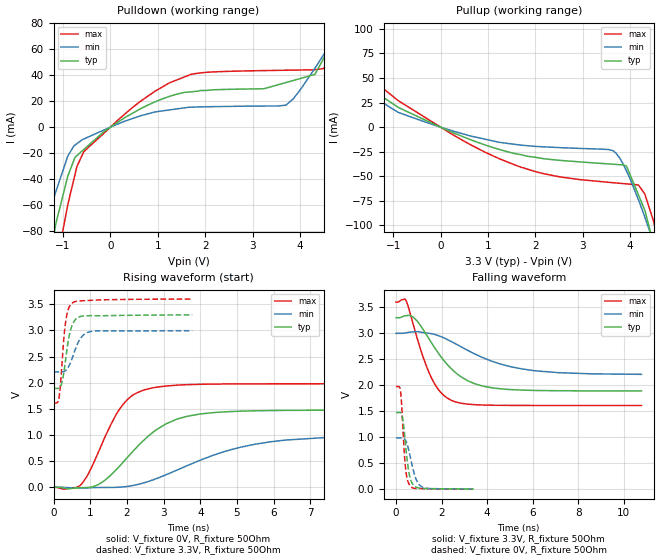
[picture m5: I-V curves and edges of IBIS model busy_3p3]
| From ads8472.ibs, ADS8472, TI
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|   busy_3p3 Model
[Model]   busy_3p3
Model_type   Output
Polarity   Non-Inverting
Vmeas = 1.65
Vref = 1.65
Cref = 5pF
Rref = 50
|   typ   min   max
|   (nom PVT)   (Fast PVT)   (slow PVT)
|C_comp from frequency method(F=1MHz)
|Average
|C_comp   8.471e-12   7.455e-12   1.492e-11
|ON state : BUFFER OUTPUT TURNED HIGH
|C_comp   8.471e-12   7.455e-12   1.492e-11
|OFF state: BUFFER OUTPUT TURNED LOW
|C_comp   5.617e-12   4.472e-12   6.741e-12
|C_comp from L-C Tank method(L=1nH)
|Resonant Frequency(Hz)   3.46e9   3.94e9   3.1e9
C_comp   2.118e-12   1.633e-12  2.638e-12
| Where nom  PVT is Nominal Process,  3.3V,  30C
|   Fast PVT is Strong Process,   3.6V,  -40C
|   Slow PVT is Weak Process,   3V,  90C
[Voltage Range]   3.3   3   3.6
|Ambient Temperature   25   85   -40
|Junction Temperature
[Temperature Range]   30   90   -40
[Pullup Reference]   3.3   3   3.6
[Pulldown Reference]   0   0   0
[Power Clamp Reference]   3.3   3   3.6
[GND Clamp Reference]   0   0   0
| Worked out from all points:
|   slope of the pulldown table from 0 to 0.495 V, typ, clamps not added: 44 ohm
|   slope of the pullup table from 0 to 0.495 V, typ, clamps not added: 48.8 ohm
|   falling waveform, V_fixture 3.3V, R_fixture 50Ohm: 20-80 % time 1.55ns typ, 2.51ns min, 984ps max; typ from 3.3 V to 1.89 V
|   rising waveform, V_fixture 0V, R_fixture 50Ohm: 20-80 % time 1.34ns typ, 2.32ns min, 849ps max; typ from 0 V to 1.48 V
|   rising waveform, V_fixture 3.3V, R_fixture 50Ohm: 20-80 % time 193ps typ, 275ps min, 144ps max; typ from 1.89 V to 3.3 V
|   falling waveform, V_fixture 0V, R_fixture 50Ohm: 20-80 % time 232ps typ, 335ps min, 168ps max; typ from 1.48 V to 0.005 V
[Pulldown]
|   Voltage   I(typ)   I(min)   I(max)
-3.3V     -554.4mA   -390.5mA   -764.5mA
-1.357V   -116.1mA   -76.09mA   -164.7mA
-1.141V   -72.84mA   -48.65mA   -106mA
-897.6mV  -37.49mA   -22.12mA   -59.52mA
-745.8mV  -23.17mA   -13.73mA   -36.37mA
-561.6mV  -17.21mA   -9.126mA   -19mA
1.246V    23.65mA    13.24mA    34.04mA
3.702V    34.28mA    16.89mA    43.81mA
4.316V    40.58mA    45.23mA    44.14mA
4.662V    63.94mA    64.84mA    54.8mA
5.28V     106.2mA    96.98mA    107.1mA
6.6V      169.4mA    151.6mA    195.9mA
[Pullup]
|   Voltage   I(typ)   I(min)   I(max)
-3.3V     137.8mA    121.9mA    160.8mA
-2.837V   119.1mA    103.6mA    142.1mA
-2.235V   90.94mA    78.66mA    107.7mA
-1.415V   40.88mA    35.74mA    47.28mA
-897mV    20.21mA    15.12mA    27.04mA
1.645V    -27.56mA   -17.98mA   -39.87mA
3.639V    -37.74mA   -24mA      -56.56mA
3.924V    -39.56mA   -44.57mA   -57.75mA
4.18V     -69.29mA   -74.17mA   -59.12mA
4.468V    -114.1mA   -113.5mA   -91.64mA
4.655V    -152.9mA   -141.4mA   -133.4mA
6.6V      -597.1mA   -466.9mA   -733.5mA
[Ramp]
R_load = 50
|   typ   min   max
dV/dt_r   0.887057/1.33633e-09   0.591584/2.32234e-09   1.18783/8.48849e-10
dV/dt_f   0.845912/1.55421e-09   0.475367/2.52494e-09   1.19342/9.8449e-10
[Falling Waveform]
V_fixture = 3.3V
V_fixture_min = 3V
V_fixture_max = 3.6V
R_fixture = 50Ohm
|   Time   V(typ)   V(min)   V(max)
0s        3.3V       3V         3.6V
430ps     3.338V     3.009V     3.639V
880ps     3.259V     3.031V     2.98V
1.19ns    3.073V     3.014V     2.544V
1.55ns    2.823V     2.993V     2.149V
1.97ns    2.552V     2.937V     1.861V
2.47ns    2.3V       2.832V     1.704V
3.65ns    2.004V     2.563V     1.623V
5.52ns    1.908V     2.316V     1.613V
10.77ns   1.891V     2.211V     1.611V
[Rising Waveform]
V_fixture = 0V
V_fixture_min = 0V
V_fixture_max = 0V
R_fixture = 50Ohm
|   Time   V(typ)   V(min)   V(max)
0s        1.018nV    1.181nV    912pV
760ps     -7.584mV   -18.63mV   59.4mV
1.25ns    63.56mV    -3.895mV   715.2mV
1.79ns    396.6mV    1.69mV     1.483V
2.13ns    661.2mV    29.56mV    1.746V
2.49ns    919.4mV    90.64mV    1.866V
3.07ns    1.214V     240.2mV    1.937V
3.64ns    1.357V     413mV      1.962V
5.9ns     1.467V     868.2mV    1.978V
10.75ns   1.477V     982.1mV    1.98V
[Rising Waveform]
V_fixture = 3.3V
V_fixture_min = 3V
V_fixture_max = 3.6V
R_fixture = 50Ohm
|   Time   V(typ)   V(min)   V(max)
0s        1.89V      2.207V     1.611V
150ps     1.894V     2.207V     1.717V
190ps     1.923V     2.206V     1.971V
240ps     2.035V     2.206V     2.456V
330ps     2.444V     2.232V     3.162V
420ps     2.87V      2.319V     3.434V
520ps     3.119V     2.491V     3.528V
740ps     3.267V     2.852V     3.564V
1.02ns    3.28V      2.978V     3.574V
3.78ns    3.296V     2.994V     3.598V
[Falling Waveform]
V_fixture = 0V
V_fixture_min = 0V
V_fixture_max = 0V
R_fixture = 50Ohm
|   Time   V(typ)   V(min)   V(max)
0s        1.477V     987.8mV    1.976V
200ps     1.475V     988.1mV    1.88V
240ps     1.452V     988.7mV    1.678V
300ps     1.341V     988.4mV    1.207V
410ps     909.3mV    949.9mV    445.4mV
480ps     606.4mV    878.8mV    224.9mV
610ps     236.9mV    658.2mV    71.75mV
870ps     43.2mV     206.6mV    16.54mV
1.16ns    16.81mV    42.14mV    13.2mV
3.41ns    5.31mV     6.83mV     2.848mV
